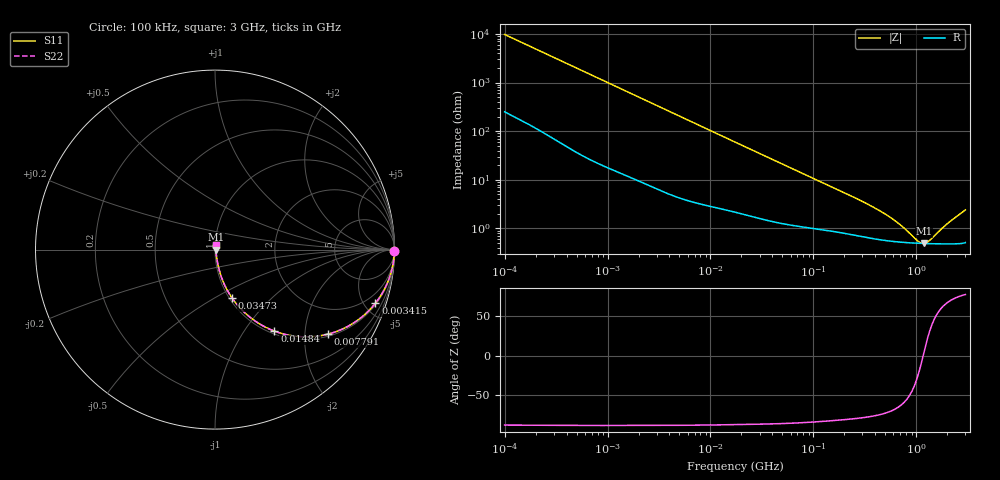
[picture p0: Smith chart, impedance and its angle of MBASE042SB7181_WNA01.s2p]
! MBASE042SB7181_WNA01  S-PARAMETER MODEL  ( Standard Model )
! Model Generated by TAIYO YUDEN Corporation (https://www.yuden.co.jp/en/)
! Version 1.0
! TAIYO YUDEN Control No. 250312
! Copyright(c) 2025 TAIYO YUDEN CO.,LTD. All Rights Reserved.
! Product Description (link to TY-COMPAS)
! https://ds.yuden.co.jp/TYCOMPAS/or/detail?pn=MBASE042SB7181KWNA01&u=M
! Products Name : Multilayer Ceramic Capacitors
! Characteristics :
!  Capacitance : 180 [pF] , Rated Voltage : 16 [V] , TCC : X7R
!  Case Size : 0.4 x 0.2 / 0.016 x 0.008 [mm/inch] , Thickness : 0.2 / 0.008 [mm/inch]
!  (Conditions: Temperature = 25 [degC] , DC Bias Voltage = 0 [V])
! External Node Assignments :
!  1  o---| |---o  2
! GND o---------o GND
! Frequency Range : 100kHz  -  3GHz  [ 401 STEP ]
# MHZ S RI R 50
! Freq[MHz].  S11 Real  S11 Imag  S21 Real  S21 Imag  S12 Real  S12 Imag  S22 Real  S22 Imag
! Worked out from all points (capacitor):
!   401 points, 100 kHz to 3 GHz, reference 50 ohm
!   read as one part in series: C = 163 pF near 105.3 kHz
!   lowest |Z| = 491 mohm at 1.186 GHz (marker M1)
!   series resonance near 1.166 GHz, so ESL is about 110 pH
!   S11 on the Smith chart (normalised r, x): 100 kHz: open; 3.415 MHz: 1.11, -5.95; 7.791 MHz: 1.06, -2.63; 14.84 MHz: 1.05, -1.39; 34.73 MHz: 1.03, -0.60; 3 GHz: 1.01, +0.05
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0.1  0.9996 -0.0102  0.000368 0.0102  0.000368 0.0102  0.9996 -0.0102
0.562235  0.9958 -0.056  0.00416 0.056  0.00416 0.056  0.9958 -0.056
1.421866  0.978 -0.1378  0.022 0.1378  0.022 0.1378  0.978 -0.1378
3.161081  0.9072 -0.2807  0.0928 0.2807  0.0928 0.2807  0.9072 -0.2807
3.415183  0.8939 -0.2984  0.1061 0.2984  0.1061 0.2984  0.8939 -0.2984
5.158208  0.7914 -0.396  0.2086 0.396  0.2086 0.396  0.7914 -0.396
7.79083  0.6301 -0.4707  0.3699 0.4707  0.3699 0.4707  0.6301 -0.4707
10.61445  0.484 -0.4857  0.516 0.4857  0.516 0.4857  0.484 -0.4857
14.83897  0.3315 -0.4543  0.6685 0.4543  0.6685 0.4543  0.3315 -0.4543
17.7727  0.2611 -0.4214  0.7389 0.4214  0.7389 0.4214  0.2611 -0.4214
24.84619  0.1599 -0.346  0.8401 0.346  0.8401 0.346  0.1599 -0.346
34.73492  0.0946 -0.2691  0.9054 0.2691  0.9054 0.2691  0.0946 -0.2691
53.83243  0.0477 -0.1843  0.9523 0.1843  0.9523 0.1843  0.0477 -0.1843
97.38194  0.0214 -0.1059  0.9786 0.1059  0.9786 0.1059  0.0214 -0.1059
294.964  0.00799 -0.0353  0.992 0.0353  0.992 0.0353  0.00799 -0.0353
547.5153  0.00574 -0.0163  0.9943 0.0163  0.9943 0.0163  0.00574 -0.0163
726.971  0.00525 -0.00969  0.9947 0.00969  0.9947 0.00969  0.00525 -0.00969
1042.837  0.00493 -0.00223  0.9951 0.00223  0.9951 0.00223  0.00493 -0.00223
1186.261  0.00487 0.000338  0.9951 -0.000338  0.9951 -0.000338  0.00487 0.000338
1349.411  0.00484 0.00292  0.9952 -0.00292  0.9952 -0.00292  0.00484 0.00292
1986.261  0.0049 0.0112  0.9951 -0.0112  0.9951 -0.0112  0.0049 0.0112
3000  0.00563 0.0233  0.9944 -0.0233  0.9944 -0.0233  0.00563 0.0233
